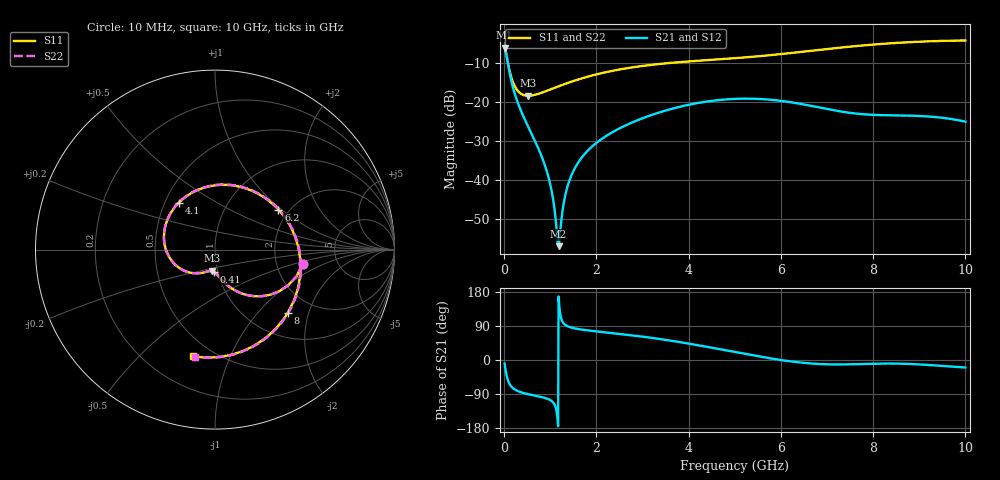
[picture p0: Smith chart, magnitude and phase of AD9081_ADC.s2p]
! Created Tue Jun 16 16:20:14 2020
# hz S ma R 50
! 2 Port Network Data from SP1.SP block
! freq  magS11  angS11  magS21  angS21  magS12  angS12  magS22  angS22
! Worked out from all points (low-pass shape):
!   1000 points, 10 MHz to 10 GHz, reference 50 ohm
!   highest |S21| = -6.16 dB at 10 MHz (marker M1); lowest = -56.9 dB at 1.18 GHz (marker M2)
!   |S21| within 3 dB of the highest: start of sweep to 63.99 MHz
!   lowest |S11| = -18.5 dB at 520 MHz (marker M3), VSWR 1.27, Z = 47.2 - j11.3 ohm
!   |S11| at or under -10 dB: 80.52 MHz to 3.688 GHz (3.608 GHz wide, 191 % of centre)
!   |S22| runs from -18.5 to -4.3 dB; largest |S21 - S12| = 0
!   S11 on the Smith chart (normalised r, x): 10 MHz: 2.82, -0.59; 410 MHz: 0.96, -0.24; 4.1 GHz: 0.59, +0.35; 6.2 GHz: 1.77, +0.95; 8 GHz: 1.49, -1.47; 10 GHz: 0.39, -0.74
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1e7  0.4949 -9.3  0.4921 -9.2  0.4921 -9.2  0.4948 -9.3
8e7  0.3174 -53.6  0.3068 -52.8  0.3068 -52.8  0.3171 -53.7
1.5e8  0.2101 -70.8  0.1898 -69.2  0.1898 -69.2  0.2099 -70.9
2.6e8  0.1471 -82.8  0.1116 -79.8  0.1116 -79.8  0.147 -83.0
4.1e8  0.1225 -92.2  0.0664 -86.8  0.0664 -86.8  0.1224 -92.3
5.2e8  0.1192 -97.5  0.04812 -90.2  0.04812 -90.2  0.1191 -97.6
9.4e8  0.1389 -114.6  0.01208 -102.5  0.01208 -102.5  0.1389 -114.6
1.04e9  0.1464 -118.4  0.006732 -109.2  0.006732 -109.2  0.1464 -118.4
1.14e9  0.1543 -122.0  0.002235 -137.9  0.002235 -137.9  0.1543 -122.1
1.18e9  0.1575 -123.5  0.001432 167.4  0.001432 167.4  0.1575 -123.5
1.38e9  0.1739 -130.7  0.008521 88.8  0.008521 88.8  0.174 -130.7
1.68e9  0.1985 -141.4  0.01931 80.3  0.01931 80.3  0.1986 -141.4
2.31e9  0.2456 -163.8  0.03966 71.5  0.03966 71.5  0.2459 -163.8
3.34e9  0.3024 158.1  0.07226 56.0  0.07226 56.0  0.3032 158.1
4.1e9  0.3303 127.4  0.09398 41.2  0.09398 41.2  0.3316 127.5
5.01e9  0.36 87.3  0.1088 20.8  0.1088 20.8  0.3619 87.5
6.2e9  0.4177 32.2  0.09886 -3.5  0.09886 -3.5  0.4199 32.7
6.67e9  0.4482 11.3  0.08826 -9.3  0.08826 -9.3  0.4504 11.9
8e9  0.5368 -41.1  0.06801 -9.7  0.06801 -9.7  0.5384 -40.3
8.34e9  0.5556 -52.7  0.06713 -9.3  0.06713 -9.3  0.5571 -51.9
9.16e9  0.5896 -78.3  0.06503 -12.8  0.06503 -12.8  0.5908 -77.4
1e10  0.606 -101.6  0.05569 -19.9  0.05569 -19.9  0.6071 -100.6
